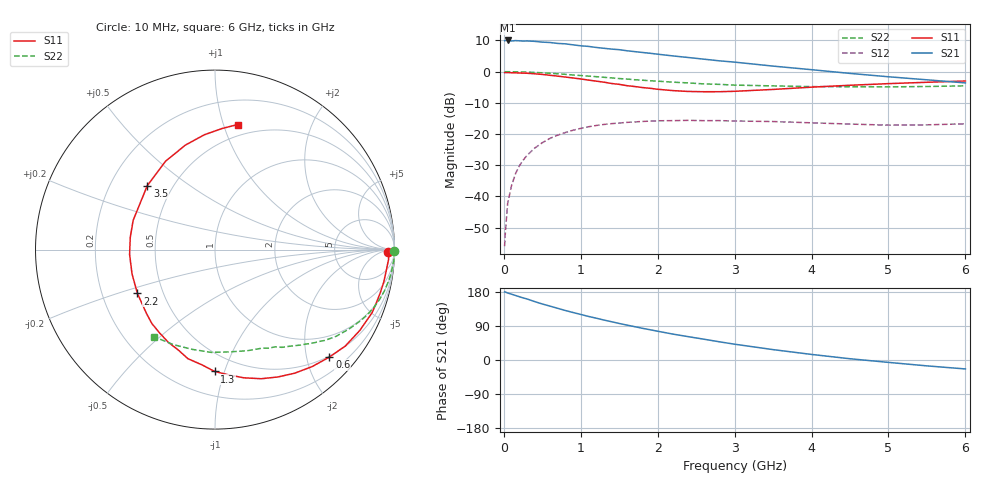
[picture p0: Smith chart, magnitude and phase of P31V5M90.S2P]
! SIEMENS Small Signal Semiconductors
! BFP181
! Si NPN RF Bipolar Junction Transistor in SOT143
! VCE = 1.5 V  IC = 0.9 mA
! Common Emitter S-Parameters:  March  1996
# GHz  S  MA  R  50
!  f  S11  S21  S12  S22
! GHz  MAG  ANG  MAG  ANG  MAG  ANG  MAG  ANG
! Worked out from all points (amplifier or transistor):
!   36 points, 10 MHz to 6 GHz, reference 50 ohm
!   highest |S21| = 10.0 dB at 50 MHz (marker M1)
!   |S21| within 3 dB of that: start of sweep to 1.513 GHz
!   unconditionally stable (mu >= 1): 3.103 GHz to end of sweep
!   at 250 MHz: K = 0.09, MSG = 19.1 dB, |S12| = -28.4 dB
!   at 1.4 GHz: K = 0.50, MSG = 11.9 dB, |S12| = -16.7 dB
!   at 6 GHz: K = 1.33, MAG = 3.1 dB, |S12| = -16.7 dB
!   S11 on the Smith chart (normalised r, x): 10 MHz: 48, -22; 600 MHz: 0.48, -2.44; 1.3 GHz: 0.37, -0.93; 2.2 GHz: 0.36, -0.23; 3.5 GHz: 0.36, +0.35; 6 GHz: 0.40, +1.12
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0.01  0.9662 -0.9  3.127 179.7  0.0016 84.7  0.9994 -0.3
0.02  0.9684 -1.5  3.157 179.4  0.0027 81.9  0.9972 -0.7
0.05  0.9684 -3.3  3.16 176.8  0.0078 89.2  0.997 -1.8
0.1  0.9609 -7.3  3.099 173.7  0.0149 83.8  0.9984 -3.5
0.15  0.9574 -11.0  3.143 170.4  0.0229 81.8  0.9932 -5.2
0.2  0.9516 -14.7  3.12 167.1  0.0307 80.2  0.9914 -6.9
0.3  0.9432 -21.9  3.104 161.2  0.0454 75.2  0.9823 -10.4
0.4  0.9239 -29.2  3.058 154.2  0.0594 70.5  0.9713 -13.8
0.6  0.8745 -43.2  2.931 142.2  0.0853 61.1  0.9419 -20.0
0.8  0.8193 -57.2  2.79 130.6  0.1059 52.9  0.9053 -25.7
1.1  0.7327 -77.2  2.537 115.0  0.1309 41.8  0.8478 -33.1
1.3  0.6787 -90.2  2.368 105.5  0.1425 35.0  0.812 -37.5
1.5  0.6264 -103.9  2.249 96.4  0.1503 29.5  0.775 -41.3
1.8  0.5567 -124.0  2.03 83.7  0.1592 22.5  0.7294 -46.2
2.2  0.4965 -150.5  1.785 68.3  0.164 14.1  0.6784 -52.6
2.8  0.477 171.9  1.491 48.1  0.1644 4.8  0.6258 -61.4
3  0.4843 160.3  1.421 41.7  0.1617 2.3  0.6084 -64.5
3.5  0.5189 136.6  1.227 27.4  0.1588 -1.9  0.5914 -72.3
4  0.5643 119.2  1.075 14.7  0.1514 -5.1  0.5758 -81.6
4.5  0.6052 105.8  0.937 3.3  0.1446 -7.2  0.5731 -92.0
5.5  0.6757 86.7  0.74 -15.5  0.1406 -3.7  0.5781 -113.7
6  0.7083 79.7  0.66 -23.6  0.1458 -2.5  0.5921 -124.8
